FUNCTION_BLOCK FB_Axis
VAR_OUTPUT
	// =============== State variables ========================
	bError							: BOOL;					// Error signal
	nErrorID						: UDINT;				// Error ID
	bMoves							: BOOL;					// Status of moving
END_VAR
VAR	
	// =============== Done signals of Halt and Reset =========
	bResetDone						: BOOL;					// Status of function block MC_Reset
	bHaltDone						: BOOL;					// Status of function block MC_Halt

	// =============== State variables ========================
	bStatusEnable					: BOOL;					// Enable feedback
	
	// =============== Velocity, override =====================
	fVelocity						: LREAL;				// Target velocity
	fOverride 						: LREAL := 100.0;		// Override 100%
	
	// =============== Trigger function blocks ================
	fbTriggerHalt					: R_TRIG;				// Trigger to recognize rising edge of halt input
	fbTriggerReset					: R_TRIG;				// Trigger to recognize rising edge of reset input
	
	// =============== Axis reference =========================
	AxisRef							: AXIS_REF;				// Axis reference (process data plc/nc)
	
	// =============== Motion function blocks =================
	fbMcPower 						: MC_Power;				// FB for enable and override
	fbMcReset 						: MC_Reset;				// FB to reset axis
	fbMcStop 						: MC_Stop;				// FB to stop axis
	fbMcHalt						: MC_Halt;				// FB to halt axis
	fbMcMove						: MC_MoveVelocity;		// FB to move axis (velocity movement)	

END_VAR

// =========================================================
;
// =========================================================

PROPERTY bState_Enable : BOOL
GET
bState_Enable := bStatusEnable;
END_GET
END_PROPERTY

PROPERTY bState_HaltDone : BOOL
GET
bState_HaltDone := bHaltDone;
END_GET
END_PROPERTY

PROPERTY bState_ResetDone : BOOL
GET
bState_ResetDone := bResetDone;
END_GET
END_PROPERTY

METHOD PUBLIC CylicCheck
VAR_INPUT
END_VAR
AxisRef.ReadStatus();
END_METHOD

METHOD Enable
VAR_INPUT
	bEnable		: BOOL;
END_VAR
// =========================================================

fbMCPower(	Enable 			:= bEnable, 
			Enable_Positive	:= bEnable, 
			Enable_Negative	:= bEnable, 
			Override		:= fOverride,
			Axis			:= AxisRef,
			Status			=> bStatusEnable,
            Error           => bError,
            ErrorID         => nErrorID);
			




bMoves := AxisRef.Status.Moving;

// =========================================================
END_METHOD

PROPERTY fTargetVelocity : LREAL
GET
fTargetVelocity := fVelocity;
END_GET
SET
fVelocity := fTargetVelocity;
END_SET
END_PROPERTY

METHOD Halt
VAR_INPUT
	bDriveHalt		: BOOL;					// Request stop
END_VAR
// =========================================================


IF bDriveHalt THEN
	fbMCMove(	Execute	:= FALSE,  Axis := AxisRef);
	fbMcHalt(	Execute	:= TRUE, 
                Axis 	:= AxisRef,
                Error   => bError,
				Done    => bHaltDone,
                ErrorID => nErrorID);
ELSIF fbMcHalt.Done OR fbMcHalt.Error OR fbMcHalt.CommandAborted THEN
	fbMcHalt(	Execute	:= FALSE,
				Axis 	:= AxisRef);
END_IF

bHaltDone:= fbMcHalt.Done AND  bDriveHalt;




// =========================================================
END_METHOD

METHOD MoveBw
VAR_INPUT
END_VAR
// =========================================================



// Not error
IF NOT (fbMcMove.Error AND fbMCMove.CommandAborted) THEN
	fbMCMove(	Execute 	:= TRUE,
				Velocity 	:= fVelocity,
				Direction 	:= MC_Negative_Direction,
				Axis 		:= AxisRef,
                Error       => bError,
                ErrorID     => nErrorID );
ELSE
		fbMCMove(	Execute	:= FALSE,
				Axis 	:= AxisRef);
END_IF



// =========================================================
END_METHOD

METHOD MoveFw
VAR_INPUT
END_VAR
// =========================================================

// Not error
IF NOT (fbMcMove.Error AND fbMCMove.CommandAborted) THEN
	fbMCMove(	Execute 	:= TRUE,
				Velocity 	:= fVelocity,
				Direction 	:= MC_Positive_Direction,
				Axis 		:= AxisRef,
                Error       => bError,
                ErrorID     => nErrorID );
ELSE
		fbMCMove(	Execute	:= FALSE,
				Axis 	:= AxisRef);
END_IF

// =========================================================
END_METHOD

METHOD Reset
VAR_INPUT
	bDriveReset		: BOOL;					// Request reset
END_VAR
// =========================================================
IF bDriveReset THEN
	fbMcReset(	Execute	:= TRUE, 
                Axis 	:= AxisRef,
                Error   => bError,
                ErrorID => nErrorID);
ELSIF fbMcReset.Done OR fbMcReset.Error  THEN
	fbMcReset(	Execute	:= FALSE,
				Axis 	:= AxisRef);
END_IF

bResetDone:= fbMcReset.Done AND bDriveReset;

// =========================================================
END_METHOD

END_FUNCTION_BLOCK
